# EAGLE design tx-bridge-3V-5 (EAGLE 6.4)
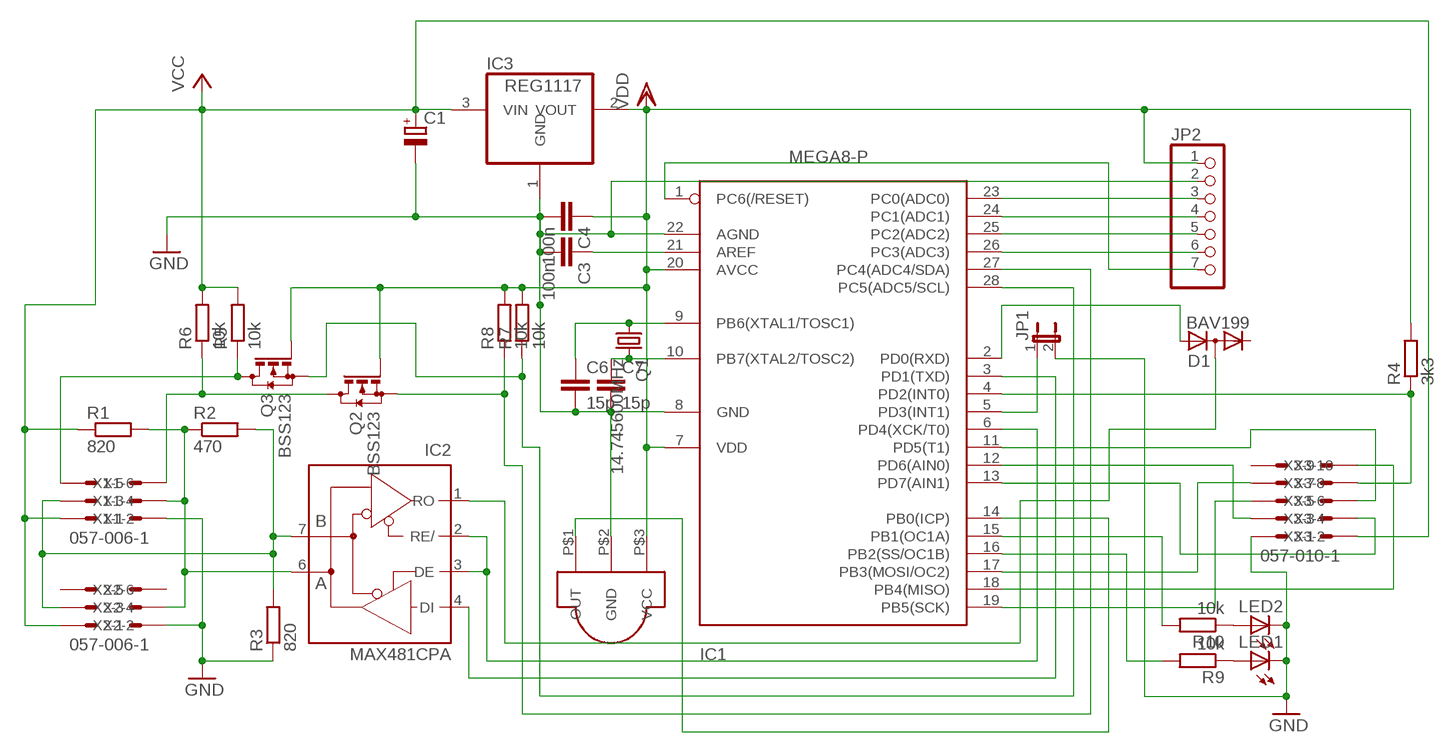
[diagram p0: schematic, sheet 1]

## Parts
C1  CPOL-EUD/7343-31R  [D/7343-31R]
C3  100n  C-EUC0805  [C0805]
C4  100n  C-EUC0805  [C0805]
C6  15p  C-EUC0805  [C0805]
C7  15p  C-EUC0805  [C0805]
D1  BAV199  [SOT23]
IC1  MEGA8-P  [DIL28-3]
IC2  MAX481CPA  [DIL08]
IC3  REG1117  [SOT223]
JP1  JP1E  [JP1]
JP2  PINHD-1X7  [1X07]
LED1  LED3MM  [LED3MM]
LED2  LED3MM  [LED3MM]
Q1  14.745600MHz  CRYSTALHC49S  [HC49/S]
Q2  BSS123  [SOT23]
Q3  BSS123  [SOT23]
R1  820  R-EU_R0805  [R0805]
R2  470  R-EU_R0805  [R0805]
R3  820  R-EU_R0805  [R0805]
R4  3k3  R-EU_R0805  [R0805]
R5  10k  R-EU_R0805  [R0805]
R6  10k  R-EU_R0805  [R0805]
R7  10k  R-EU_R0805  [R0805]
R8  10k  R-EU_R0805  [R0805]
R9  10k  R-EU_R0805  [R0805]
R10  10k  R-EU_R0805  [R0805]
U$1  SFH5110-XX  [SFH5110-XX]
X1  057-006-1  [057-006-1]
X2  057-006-1  [057-006-1]
X3  057-010-1  [057-010-1]

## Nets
GND: C1.- C3.2 C4.2 C6.2 C7.2 IC1.8(GND) IC1.22(AGND) IC3.1(GND) JP1.2 JP2.2 LED1.K(C) LED2.K(C) R3.1 U$1.P$2(GND) X1.1 X2.1 X3.2
N$1: IC1.16(PB2(SS/OC1B)) R9.2
N$2: IC1.15(PB1(OC1A)) R10.2
N$3: LED1.A R9.1
N$4: IC1.17(PB3(MOSI/OC2)) X3.8
N$5: IC2.7(B) R2.2 R3.2 X1.4 X2.4
N$6: LED2.A R10.1
N$7: IC2.6(A) R1.2 R2.1 X1.3 X2.3
N$8: C7.1 IC1.10(PB7(XTAL2/TOSC2)) Q1.2
N$9: C6.1 IC1.9(PB6(XTAL1/TOSC1)) Q1.1
N$10: IC1.4(PD2(INT0)) R4.1 X3.7
N$11: IC1.26(PC3(ADC3)) JP2.6
N$12: IC1.6(PD4(XCK/T0)) IC2.2(RE/) IC2.3(DE)
N$13: IC1.3(PD1(TXD)) IC2.4(DI)
N$14: D1.3(AC) IC2.1(RO)
N$15: IC1.27(PC4(ADC4/SDA)) Q2.2(S) R8.1
N$16: IC1.28(PC5(ADC5/SCL)) Q3.2(S) R7.1
N$17: C3.1 IC1.21(AREF)
N$18: IC1.19(PB5(SCK)) X3.6
N$19: IC1.12(PD6(AIN0)) X3.4
N$20: IC1.25(PC2(ADC2)) JP2.5
N$21: IC1.24(PC1(ADC1)) JP2.4
N$22: IC1.23(PC0(ADC0)) JP2.3
N$24: IC1.13(PD7(AIN1)) X3.3
N$25: IC1.11(PD5(T1)) X3.5
N$26: IC1.18(PB4(MISO)) X3.9
N$27: IC1.5(PD3(INT1)) JP1.1
N$28: Q3.3(D) R5.1 X1.6
N$29: Q2.3(D) R6.1 X1.5
N$30: D1.1(A) IC1.2(PD0(RXD))
N$31: IC1.14(PB0(ICP)) U$1.P$1(OUT)
N$32: IC1.1(PC6(/RESET)) JP2.7
VCC: C1.+ IC3.3(VIN) R1.1 R5.2 R6.2 X1.2 X2.2 X3.1
VDD: C4.1 IC1.7(VDD) IC1.20(AVCC) IC3.2(VOUT) JP2.1 Q2.1(G) Q3.1(G) R4.2 R7.2 R8.2 U$1.P$3(VCC)
Unconnected: D1.2(C) X2.5 X2.6 X3.10

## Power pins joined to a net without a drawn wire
GND: IC2.5(GND)
VCC: IC2.8(VCC)

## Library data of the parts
C1 = rcl:CPOL-EU: POLARIZED CAPACITOR, European symbol
C3 C4 C6 C7 = rcl:C-EU: CAPACITOR, European symbol
D1 = diode:BAV199: DIODE low-leakage double diode
IC1 = atmel:MEGA8-P: MICROCONTROLLER 8 Kbytes FLASH, 1 kbytes SRAM, 512 bytes EEPROM, USART, 4-channel 10 bit ADC, 2-channel 8 bit ADC Pin compatible with Atmega48, ATMega88, ATMega168 Source: avr.lbr
IC2 = maxim:MAX481CPA: RS485 TRANSEIVER; MPN: MAX481CPA+; OC_FARNELL: unknown; OC_NEWARK: 99K3445
IC3 = burr-brown:REG1117: 800mA and 1A Low Dropout (LDO) Positive Regulator 1.8V, 2.5V, 2.85V, 3.3V, 5V, and Adj; MPN: REG1117; OC_FARNELL: 1097566; OC_NEWARK: 14P6981
JP1 = jumper:JP1E: JUMPER
JP2 = pinhead:PINHD-1X7: PIN HEADER
LED1 LED2 = led:LED: LED
Q1 = crystal:CRYSTAL: CRYSTAL
Q2 Q3 = transistor-small-signal:BSS123: N-CHANNEL MOS FET
R1-R10 = rcl:R-EU_: RESISTOR, European symbol
U$1 = myown:SFH5110-XX
X1 X2 = con-panduit:057-006-: CONNECTOR 6-pin series 057 contact pc board low profile headers; OC_FARNELL: unknown; OC_NEWARK: unknown
X3 = con-panduit:057-010-: CONNECTOR 10-pin series 057 contact pc board low profile headers; OC_FARNELL: unknown; OC_NEWARK: unknown

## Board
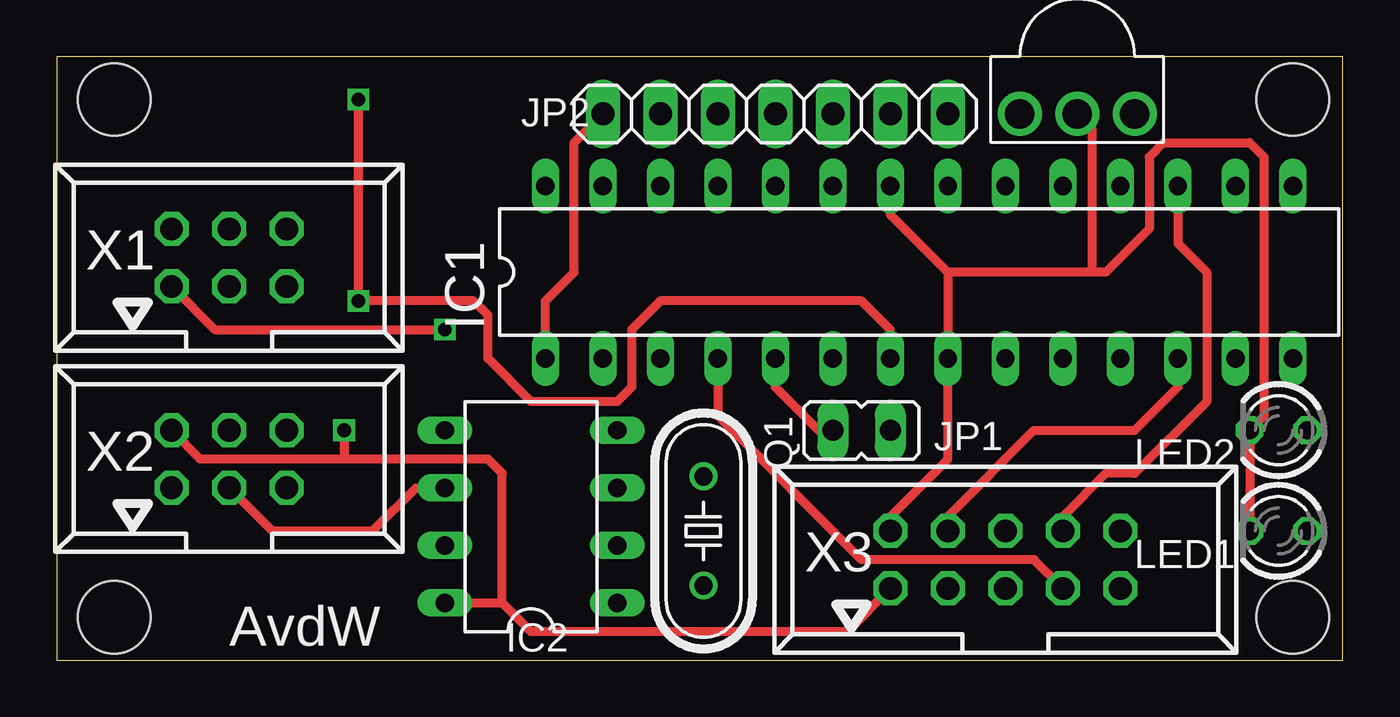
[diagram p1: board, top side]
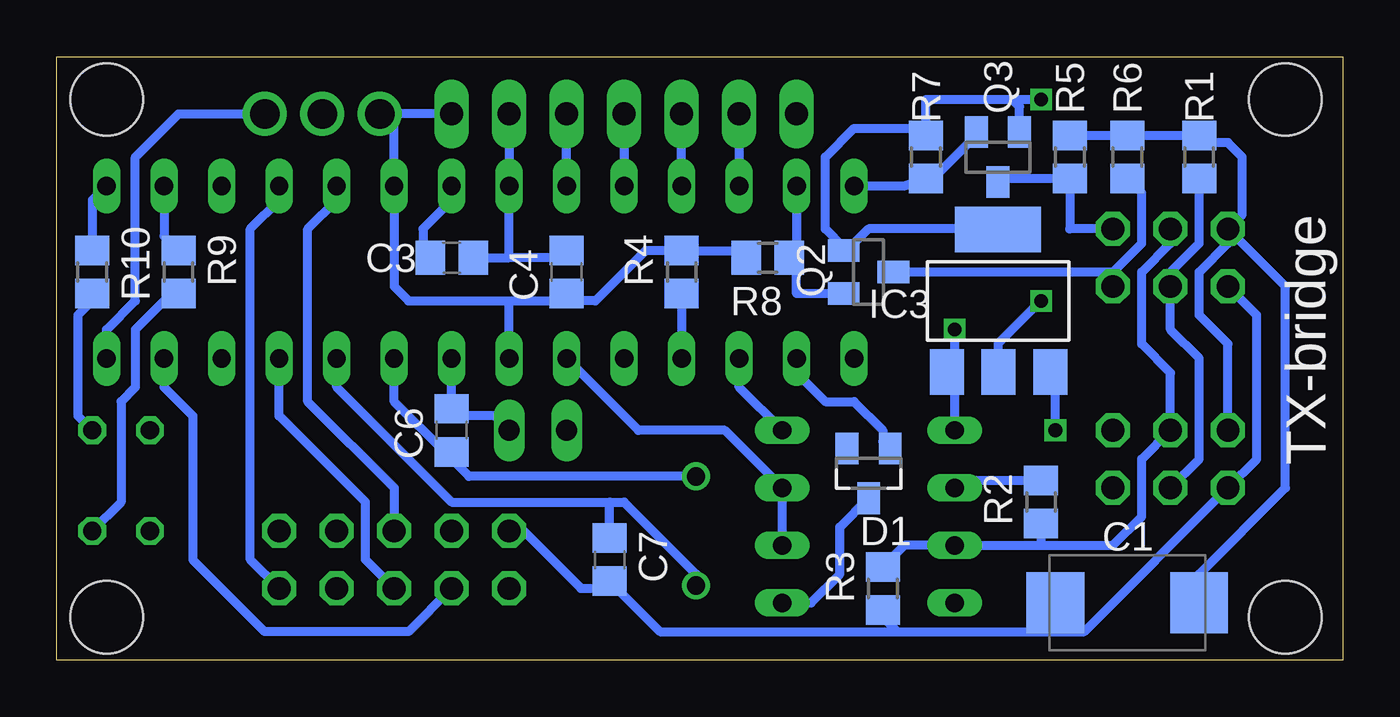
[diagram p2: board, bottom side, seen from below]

Size 56.82 x 26.66 mm. Coordinates in mm from the lower left corner, seen from the top.
Outline: 0,0 56.82,0 56.82,26.66 0,26.66 0,0
Copper layers (1*16): Top 0.0356mm / dielectric 1.5011mm / Bottom 0.0356mm
Design rules "oshpark": minimum track width 6mil, minimum drill 13mil, track to track 6mil, track to pad 6mil, pad to pad 6mil, via to via 6mil, smd to smd 6mil, copper to edge 15mil, drill to drill 6mil, minimum pad ring 7mil, minimum via ring 7mil, stop-mask expansion 3mil, vias tented up to drill 0mil, thermal gap 10mil
Holes 3.2 mm at 2.54,1.91 54.61,24.77 54.61,1.91 2.54,24.77

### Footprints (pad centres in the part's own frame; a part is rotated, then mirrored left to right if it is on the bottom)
D/7343-31R = smd 2.55 x 2.7: + 3.175,0; - -3.175,0
C0805 = smd 1.3 x 1.5: 1 -0.95,0; 2 0.95,0
SOT23 = smd 1 x 1.4: 1 -0.95,-1.1; 2 0.95,-1.1; 3 0,1.1
DIL28-3 = drill 0.813 long: 1 -16.51,-3.81; 2 -13.97,-3.81; 3 -11.43,-3.81; 4 -8.89,-3.81; 5 -6.35,-3.81; 6 -3.81,-3.81; 7 -1.27,-3.81; 8 1.27,-3.81; 9 3.81,-3.81; 10 6.35,-3.81; 11 8.89,-3.81; 12 11.43,-3.81; 13 13.97,-3.81; 14 16.51,-3.81; 15 16.51,3.81; 16 13.97,3.81; 17 11.43,3.81; 18 8.89,3.81; 19 6.35,3.81; 20 3.81,3.81; 21 1.27,3.81; 22 -1.27,3.81; 23 -3.81,3.81; 24 -6.35,3.81; 25 -8.89,3.81; 26 -11.43,3.81; 27 -13.97,3.81; 28 -16.51,3.81
DIL08 = drill 0.813 long: 1 -3.81,-3.81; 2 -1.27,-3.81; 3 1.27,-3.81; 4 3.81,-3.81; 5 3.81,3.81; 6 1.27,3.81; 7 -1.27,3.81; 8 -3.81,3.81
SOT223 = smd 1.499 x 2.007: 1 -2.261,-3.15; 2 0.025,-3.15; 3 2.311,-3.15 | smd 3.81 x 2.007: 4 0,3.15
JP1 = drill 0.914 long: 1 0,-1.27; 2 0,1.27
1X07 = drill 1.016 long: 1 -7.62,0; 2 -5.08,0; 3 -2.54,0; 4 0,0; 5 2.54,0; 6 5.08,0; 7 7.62,0
LED3MM = drill 0.813 octagon: A -1.27,0; K 1.27,0
HC49/S = drill 0.813: 1 -2.413,0; 2 2.413,0
R0805 = smd 1.3 x 1.5: 1 -0.95,0; 2 0.95,0
SFH5110-XX = drill 1.3: P$1 0,2.54; P$2 0,0; P$3 0,-2.54
057-006-1 = drill 1 octagon: 1 -2.54,-1.27; 2 -2.54,1.27; 3 0,-1.27; 4 0,1.27; 5 2.54,-1.27; 6 2.54,1.27
057-010-1 = drill 1 octagon: 1 -5.08,-1.27; 2 -5.08,1.27; 3 -2.54,-1.27; 4 -2.54,1.27; 5 0,-1.27; 6 0,1.27; 7 2.54,-1.27; 8 2.54,1.27; 9 5.08,-1.27; 10 5.08,1.27

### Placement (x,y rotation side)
C1  9.53,2.54 0 bottom
C3  39.37,17.78 0 bottom
C4  34.29,17.14 90 bottom
C6  39.37,10.16 90 bottom
C7  32.38,4.45 270 bottom
D1  20.95,8.26 180 bottom
IC1  38.1,17.14 0 top
IC2  20.95,6.35 90 top
IC3  15.24,15.88 0 bottom
JP1  35.56,10.16 270 top
JP2  31.75,24.13 180 top
LED1  53.98,5.71 180 top
LED2  53.98,10.16 180 top
Q1  28.57,5.71 270 top
Q2  20.95,17.14 270 bottom
Q3  15.24,22.23 180 bottom
R1  6.35,22.23 270 bottom
R2  13.34,6.99 270 bottom
R3  20.32,3.17 90 bottom
R4  29.21,17.14 90 bottom
R5  12.06,22.23 90 bottom
R6  9.53,22.23 90 bottom
R7  18.41,22.23 90 bottom
R8  25.4,17.78 180 bottom
R9  51.44,17.14 90 bottom
R10  55.24,17.14 90 bottom
U$1  45.09,24.13 270 top
X1  7.62,17.78 0 top
X2  7.62,8.89 0 top
X3  41.91,4.45 0 top

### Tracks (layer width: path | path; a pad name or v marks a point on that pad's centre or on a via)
GND  (via drill 0.6)
  Top 0.406: 39.37,17.14 IC1.8 39.37,8.89 36.83,6.35 X3.2 | X1.1 6.99,14.61 v17.14,14.61 | LED1.K LED2.K 53.34,10.79 53.34,22.23 52.7,22.86 48.9,22.86 48.26,22.23 48.26,19.05 46.35,17.14 45.72,17.14 | 45.72,17.14 39.37,17.14 | 39.37,17.14 36.83,19.68 IC1.22 | U$1.P$2 45.72,23.5 45.72,17.14
  Bottom 0.406: X1.1 3.81,15.24 3.81,8.89 X2.1 11.43,1.27 12.7,1.27 | 36.83,17.78 IC1.22 JP2.2 | C3.2 36.83,17.78 | X3.2 36.2,5.71 33.66,3.17 32.7,3.17 C7.2 30.16,1.27 19.68,1.27 | 19.68,1.27 12.7,1.27 | IC2.5 17.14,12.37 IC3.1 17.5,12.98 17.14,13.34 v17.14,14.61 | C4.2 34.29,17.78 36.83,17.78 | IC1.8 C6.2 39.05,10.79 37.47,10.79 JP1.2 | R3.1 20.32,1.91 19.68,1.27 | C1.- 12.7,1.27
N$1
  Bottom 0.406: IC1.16 52.07,18.73 R9.2
N$2
  Bottom 0.406: IC1.15 55.24,20.32 R10.2
N$3
  Bottom 0.406: R9.1 51.75,16.2 53.34,14.61 53.34,12.06 53.98,11.43 53.98,6.99 LED1.A
N$4
  Top 0.406: IC1.17 49.53,18.41 50.8,17.14 50.8,11.43 47.62,8.26 46.35,8.26 44.45,6.35 X3.8
N$5
  Bottom 0.406: X1.4 7.62,18.41 8.89,17.14 8.89,13.97 7.62,12.7 X2.4 8.89,8.89 8.89,6.35 10.16,5.08 13.34,5.08 | 13.34,5.08 IC2.7 19.36,5.08 R3.2 | R2.2 13.34,5.08
N$6
  Bottom 0.406: R10.1 55.24,15.88 55.88,15.24 55.88,10.79 LED2.A
N$7
  Top 0.406: X2.3 9.53,5.71 13.97,5.71 15.88,7.62 IC2.6
  Bottom 0.406: R1.2 6.35,18.41 7.62,17.14 X1.3 7.62,14.61 6.35,13.34 6.35,8.89 X2.3 | R2.1 16.83,7.93 IC2.6
N$8
  Bottom 0.406: IC1.10 44.45,12.06 39.37,6.99 32.38,6.99 | 32.38,6.99 31.75,6.99 28.57,3.81 Q1.2 | C7.1 32.38,6.99
N$9
  Bottom 0.406: Q1.1 38.61,8.13 39.69,9.21 | 39.69,9.21 41.91,11.43 IC1.9 | C6.1 39.69,9.21
N$10
  Top 0.406: X3.7 43.18,4.45 35.56,4.45 29.21,10.79 IC1.4
  Bottom 0.406: R4.1 IC1.4
N$11
  Bottom 0.406: JP2.6 IC1.26
N$12
  Bottom 0.406: IC2.2 IC2.3 27.3,10.16 31.11,10.16 IC1.6
N$13
  Bottom 0.406: IC2.4 26.67,12.06 IC1.3
N$14
  Bottom 0.406: IC2.1 23.5,2.54 22.23,3.81 22.23,5.88 D1.3
N$15
  Bottom 0.406: Q2.2 24.14,16.2 24.14,17.46 R8.1 24.13,18.1 IC1.27
N$16
  Bottom 0.406: Q3.2 16.19,23.18 17.78,21.59 18.09,21.59 R7.1 19.37,20.95 IC1.28
N$17
  Bottom 0.406: IC1.21 39.37,20.32 40.64,19.05 40.64,18.1 C3.1
N$18
  Bottom 0.406: IC1.19 44.45,20.32 45.72,19.05 45.72,11.43 41.91,7.62 X3.6
N$19
  Top 0.406: X3.4 39.37,6.35 43.18,10.16 47.62,10.16 49.53,12.06 IC1.12
N$20
  Bottom 0.406: IC1.25 JP2.5
N$21
  Bottom 0.406: JP2.4 IC1.24
N$22
  Bottom 0.406: IC1.23 JP2.3
N$23
  Bottom 0.406: 16.51,19.05 20.95,19.05 21.59,18.41
N$24
  Bottom 0.406: X3.3 41.27,1.27 47.62,1.27 50.8,4.45 50.8,10.79 52.07,12.06 IC1.13
N$25
  Bottom 0.406: X3.5 43.18,4.45 43.18,6.99 46.99,10.79 IC1.11
N$26
  Bottom 0.406: X3.9 48.26,4.45 48.26,19.05 46.99,20.32 IC1.18
N$27
  Top 0.406: JP1.1 33.66,10.16 31.75,12.06 IC1.5
N$28
  Bottom 0.406: X1.6 12.06,19.05 R5.1 15.09,21.27 Q3.3
N$29
  Bottom 0.406: X1.5 10.16,17.14 | 10.16,17.14 8.89,18.41 8.89,20.64 R6.1 | 10.16,17.14 Q2.3
N$30
  Bottom 0.406: IC1.2 24.13,12.7 22.86,11.43 21.59,11.43 20.32,10.16 20.32,9.67 D1.1
N$31
  Bottom 0.406: U$1.P$1 51.44,24.13 53.34,22.23 53.34,15.88 54.61,14.61 IC1.14
N$32
  Top 0.406: IC1.1 21.59,15.88 22.86,17.14 22.86,22.86 JP2.7
VCC  (via drill 0.6)
  Top 0.406: 12.7,8.89 19.05,8.89 19.68,8.26 19.68,2.54 | 12.7,8.89 6.35,8.89 X2.2 | 19.68,2.54 20.95,1.27 34.92,1.27 X3.1 | IC2.8 19.68,2.54 | v12.7,10.16 12.7,8.89
  Bottom 0.406: X2.2 5.08,13.97 6.35,15.24 6.35,17.14 5.08,18.41 X1.2 | R5.2 R6.2 R1.1 6.04,22.86 5.08,22.86 4.45,22.23 4.45,19.68 X1.2 | v12.7,10.16 12.7,12.5 IC3.3 | C1.+ 6.35,3.81 2.54,7.62 2.54,16.51 X1.2
VDD  (via drill 0.6)
  Top 0.406: v13.34,24.77 v13.34,15.88 18.41,15.88 19.05,15.24 19.05,13.34 20.95,11.43 24.77,11.43 25.4,12.06 25.4,14.61 26.67,15.88 35.56,15.88 36.83,14.61 IC1.7
  Bottom 0.406: v13.34,24.77 14.61,24.77 | 14.61,24.77 18.41,24.77 R7.2 18.73,23.5 21.59,23.5 22.86,22.23 22.86,19.05 22.05,18.25 Q2.1 | Q3.1 14.29,24.45 14.61,24.77 | 36.83,15.88 41.27,15.88 41.91,16.51 IC1.20 41.91,24.13 | IC1.7 36.83,15.88 | 36.83,15.88 34.92,15.88 34.6,16.2 C4.1 33.97,15.88 33.02,15.88 30.8,18.09 R4.2 | 28.89,18.41 R4.2 | v13.34,15.88 15.24,13.97 15.24,12.75 IC3.2 | JP2.1 41.91,24.13 | 41.91,24.13 U$1.P$3 | 26.35,18.09 R8.2 26.66,18.09 R4.2

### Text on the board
tNames: AvdW
bNames: TX-bridge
